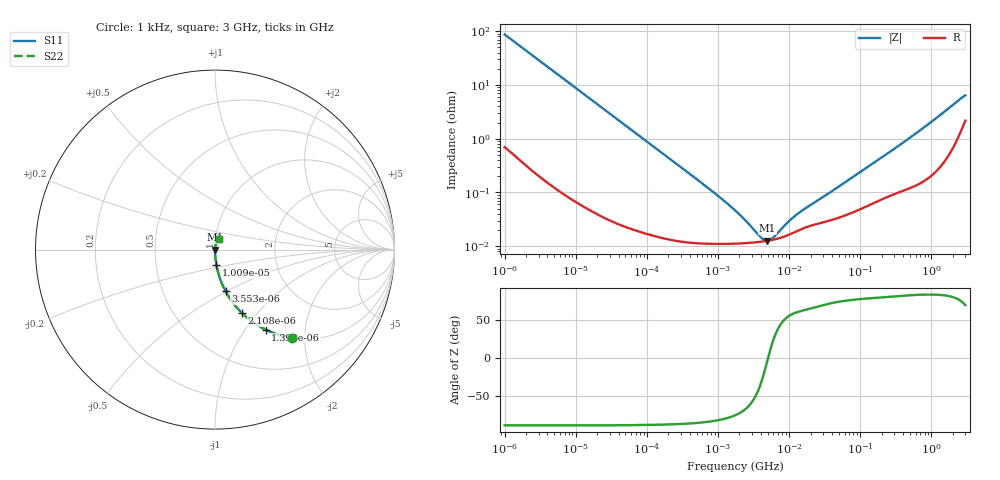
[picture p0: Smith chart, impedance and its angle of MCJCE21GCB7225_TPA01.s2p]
! MCJCE21GCB7225_TPA01  S-PARAMETER MODEL  ( Standard Model )
! Model Generated by TAIYO YUDEN Corporation (http://www.ty-top.com)
! Version 1.0
! TAIYO YUDEN Control No. 220601
! Copyright(c) 2015 TAIYO YUDEN CO.,LTD. All Rights Reserved.
! Product Description (link to TY-COMPAS)
! https://ds.yuden.co.jp/TYCOMPAS/or/detail?pn=MCJCE21GCB7225KTPA01&u=M
! Products Name : Multilayer Ceramic Capacitors
! Characteristics :
!  Capacitance : 2.2 [uF] , Rated Voltage : 16 [V] , TCC : X7R
!  Case Size : 2.0 x 1.25 / 0.079 x 0.049 [mm/inch] , Thickness : 1.25 / 0.049 [mm/inch]
!  (Conditions: Temperature = 25 [degC] , DC Bias Voltage = 0 [V])
! External Node Assignments :
!  1  o---| |---o  2
! GND o---------o GND
! Frequency Range : 1kHz  -  3GHz  [ 401 STEP ]
# MHZ S RI R 50
! Freq[MHz].  S11 Real  S11 Imag  S21 Real  S21 Imag  S12 Real  S12 Imag  S22 Real  S22 Imag
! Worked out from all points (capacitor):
!   401 points, 1 kHz to 3 GHz, reference 50 ohm
!   read as one part in series: C = 1.82 uF near 1.077 kHz
!   lowest |Z| = 12.6 mohm at 4.92 MHz (marker M1)
!   series resonance near 5.044 MHz, so ESL is about 550 pH
!   S11 on the Smith chart (normalised r, x): 1 kHz: 1.01, -1.74; 1.399 kHz: 1.01, -1.25; 2.108 kHz: 1.01, -0.83; 3.553 kHz: 1.00, -0.49; 10.09 kHz: 1.00, -0.17; 3 GHz: 1.04, +0.12
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0.001  0.4318 -0.4913  0.5682 0.4913  0.5682 0.4913  0.4318 -0.4913
0.001399  0.2816 -0.446  0.7184 0.446  0.7184 0.446  0.2816 -0.446
0.002108  0.1485 -0.352  0.8515 0.352  0.8515 0.352  0.1485 -0.352
0.003553  0.0587 -0.2317  0.9413 0.2317  0.9413 0.2317  0.0587 -0.2317
0.005768  0.0236 -0.1484  0.9764 0.1484  0.9764 0.1484  0.0236 -0.1484
0.010091  0.00818 -0.0864  0.9918 0.0864  0.9918 0.0864  0.00818 -0.0864
0.01216  0.00577 -0.0719  0.9942 0.0719  0.9942 0.0719  0.00577 -0.0719
0.033275  0.000987 -0.0265  0.999 0.0265  0.999 0.0265  0.000987 -0.0265
0.147855  0.000183 -0.00601  0.9998 0.00601  0.9998 0.00601  0.000183 -0.00601
0.762639  0.000112 -0.00114  0.9999 0.00114  0.9999 0.00114  0.000112 -0.00114
1.732051  0.000112 -0.000453  0.9999 0.000453  0.9999 0.000453  0.000112 -0.000453
2.422679  0.000114 -0.000281  0.9999 0.000281  0.9999 0.000281  0.000114 -0.000281
3.93371  0.000121 -8.71e-05  0.9999 8.71e-05  0.9999 8.71e-05  0.000121 -8.71e-05
4.399271  0.000123 -4.74e-05  0.9999 4.74e-05  0.9999 4.74e-05  0.000123 -4.74e-05
4.919932  0.000126 -8.53e-06  0.9999 8.53e-06  0.9999 8.53e-06  0.000126 -8.53e-06
5.928204  0.000132 5.57e-05  0.9999 -5.57e-05  0.9999 -5.57e-05  0.000132 5.57e-05
12.03889  0.000183 0.000316  0.9998 -0.000316  0.9998 -0.000316  0.000183 0.000316
21.06097  0.000245 0.000559  0.9998 -0.000559  0.9998 -0.000559  0.000245 0.000559
256.0921  0.000884 0.00554  0.9991 -0.00554  0.9991 -0.00554  0.000884 0.00554
783.755  0.00188 0.0161  0.9981 -0.0161  0.9981 -0.0161  0.00188 0.0161
2584.342  0.0163 0.0527  0.9837 -0.0527  0.9837 -0.0527  0.0163 0.0527
3000  0.0247 0.0576  0.9753 -0.0576  0.9753 -0.0576  0.0247 0.0576
